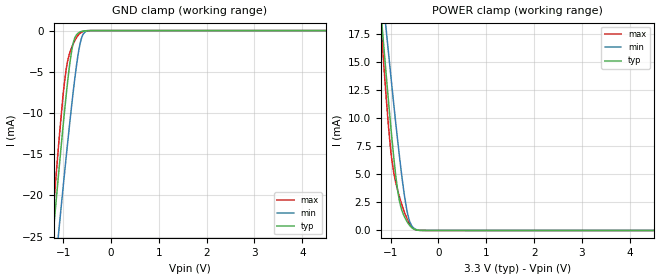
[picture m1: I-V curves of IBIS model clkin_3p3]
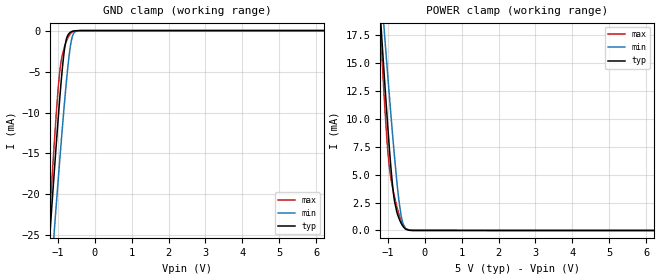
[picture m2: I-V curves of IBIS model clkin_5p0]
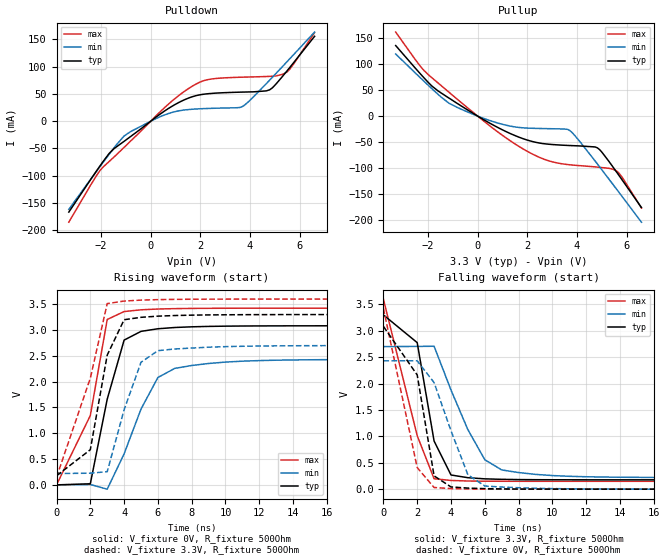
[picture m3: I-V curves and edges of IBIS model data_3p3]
| Texas Instruments Incorporated
| Small, High-Precision, Reinforced Isolated Delta-Sigma Modulator
| for Voltage Sensing Applications
| Marketing Part # : AMC3306
| Digital Voltage Range : 2.7V-5.5V
| Package-type: SOIC
| #pins/pkg drawing : 16-pin DWE
[IBIS Ver] 3.2
[File name] amc3306.ibs
[File Rev] 1.0
[Date] 08/19/2020
[Source]
| Texas Instruments Incorporated.
| 12500 TI Blvd
| Dallas, TX -75243
[Notes] Revision History:
| Rev 1.0: 08/19/2020
| - Initial version of the model
| - Model generated from simulations in SPECTRE
| - CLKIN curves from amc3306m25.ibs
| - C_comp although listed in numerical order of value are
| obtained from varying PVT conditions. For PVT conditions for
| each specific value refer the buffer description under
| respective [Model]. IBIS model user is responsible for using
| appropriate C_comp to simulate for Signal Integrity.
| - Model names with a trailing _3p3 contain the model for
| 3.3V operation. Model names with a trailing _5p0 contain the model
| for 5.0V operation.
[Disclaimer]
| This model is designed as an aid for customers of Texas Instruments.
| TI and its licensors and suppliers make no warranties, either expressed
| or implied, with respect to this model, including the warranties of
| merchantability or fitness for a particular purpose. The model is
| provided solely on an "as is" basis. The entire risk as to its quality
| and performance is with the customer.
| This model is subject to change without notice. Texas Instruments
| Incorporated is not responsible for updating this model.
[Copyright]
(C) Copyright 2020 Texas Instruments Incorporated. All rights reserved.
[Component] AMC3306
[Manufacturer] Texas Instruments Incorporated
[Package] |SOIC (DWE) 16-pin
| variable typ min max
R_pkg 0.11 0.11 0.11
L_pkg 2.9nH 2.9nH 2.9nH
C_pkg 0.4pF 0.4pF 0.4pF
| pin number (pin name) mapping to model name
[Pin]  signal_name   model_name   R_pin L_pin C_pin
1   DCDC_OUT   NC   NA   NA   NA
2   DCDC_HGND   NC   NA   NA   NA
3   HLDO_IN   NC   NA   NA   NA
4   NC   NC   NA   NA   NA
5   HLDO_OUT   NC   NA   NA   NA
6   INP   NC   NA   NA   NA
7   INN   NC   NA   NA   NA
8   HGND   NC   NA   NA   NA
9   AGND   GND   NA   NA   NA
10   DOUT   data   NA   NA   NA
11   CLKIN   clkin   NA   NA   NA
12   VDD   POWER   NA   NA   NA
13   LDO_OUT   NC   NA   NA   NA
14   DIAG   NC   NA   NA   NA
15   DCDC_GND   NC   NA   NA   NA
16   DCDC_IN   NC   NA   NA   NA
| Model Selectors
[Model Selector] clkin
clkin_3p3   3.3V digital Input
clkin_5p0   5.0V digital Input
[Model Selector] data
data_3p3   3.3V digital Output
data_5p0   5.0V digital Output
| Models and submodels in the file (4): clkin_3p3 (Input), clkin_5p0 (Input), data_3p3 (Output), data_5p0 (Output)
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|   clkin_3p3 Model
[Model]   clkin_3p3
Model_type   Input
Vinl = 0.81
Vinh = 2.52
|   typ   min   max
C_comp   1.27pF   1.27pF   1.27pF
[Voltage Range]   3.3   2.7   3.6
[Temperature Range]   25   125   -40
[Power Clamp Reference]   3.3   2.7   3.6
[GND Clamp Reference]   0   0   0
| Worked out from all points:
|   GND clamp passes 1 mA (typ) near -0.76 V on its own axis
|   POWER clamp passes 1 mA (typ) near -0.68 V on its own axis
[GND Clamp]
|   Voltage   I(typ)   I(min)   I(max)
-3.3V     -168.5mA   -163.8mA   -187mA
-1.231V   -26.22mA   -32.85mA   -23.77mA
-1.211V   -24.92mA   -31.65mA   -22.3mA
-1.092V   -17.27mA   -24.5mA    -13.76mA
-1.003V   -11.76mA   -19.24mA   -8.012mA
-933.9mV  -7.747mA   -15.26mA   -4.63mA
-815.1mV  -2.261mA   -8.782mA   -1.974mA
-745.8mV  -780uA     -5.384mA   -1.106mA
-636.9mV  -152.3uA   -1.394mA   -283.4uA
-547.8mV  -32.09uA   -196.9uA   -56.31uA
-438.9mV  -2.267uA   -11.38uA   -3.33uA
6.6V      0A         0A         0A
[POWER Clamp]
|   Voltage   I(typ)   I(min)   I(max)
-3.3V     134.4mA    118.6mA    160mA
-1.221V   20.46mA    23.51mA    19.62mA
-1.132V   15.89mA    19.63mA    14.17mA
-1.092V   13.9mA     17.92mA    11.88mA
-983.4mV  8.68mA     13.31mA    6.622mA
-884.4mV  4.605mA    9.284mA    4.137mA
-815.1mV  2.641mA    6.627mA    3.014mA
-735.9mV  1.473mA    3.887mA    1.934mA
-656.7mV  795.8uA    1.747mA    1.055mA
-597.3mV  434.4uA    769.8uA    555uA
-488.4mV  80.75uA    131.9uA    82.36uA
6.6V      0A         0A         0A
|   clkin_5p0 Model
[Model]   clkin_5p0
Model_type   Input
Vinl = 1.35
Vinh = 3.85
|   typ   min   max
C_comp   1.27pF   1.27pF   1.27pF
[Voltage Range]   5   4.5   5.5
[Temperature Range]   25   125   -40
[Power Clamp Reference]   5   4.5   5.5
[GND Clamp Reference]   0   0   0
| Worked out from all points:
|   GND clamp passes 1 mA (typ) near -0.76 V on its own axis
|   POWER clamp passes 1 mA (typ) near -0.68 V on its own axis
[GND Clamp]
|   Voltage   I(typ)   I(min)   I(max)
-5V       -287.4mA   -273.3mA   -323.4mA
-1.25V    -27.47mA   -34.01mA   -25.19mA
-1.235V   -26.49mA   -33.1mA    -24.07mA
-1.145V   -20.63mA   -27.65mA   -17.48mA
-1.1V     -17.76mA   -24.95mA   -14.3mA
-950mV    -8.649mA   -16.17mA   -5.277mA
-830mV    -2.776mA   -9.559mA   -2.198mA
-770mV    -1.136mA   -6.523mA   -1.378mA
-695mV    -365.7uA   -3.238mA   -637.9uA
-605mV    -90.88uA   -751.5uA   -166.7uA
-395mV    -749.7nA   -3.614uA   -858.5nA
10V       0A         0A         0A
[POWER Clamp]
|   Voltage   I(typ)   I(min)   I(max)
-5V       319.9mA    231.9mA    422.9mA
-1.25V    21.97mA    24.79mA    21.45mA
-1.13V    15.79mA    19.55mA    14.06mA
-1.085V   13.54mA    17.61mA    11.48mA
-995mV    9.213mA    13.8mA     7.066mA
-935mV    6.564mA    11.32mA    5.171mA
-830mV    2.979mA    7.184mA    3.241mA
-725mV    1.364mA    3.549mA    1.802mA
-635mV    651.4uA    1.322mA    855.8uA
-575mV    330.5uA    547.9uA    411.1uA
-500mV    101.7uA    162.3uA    107.5uA
10V       0A         0A         0A
|   data_3p3 Model
[Model]   data_3p3
Model_type   Output
Polarity   Non-Inverting
Vmeas = 1.65
Vref = 0
Cref = 2pF
Rref = 100000
|   typ   min   max
|   (nom PVT)   (fast PVT)   (slow PVT)
C_comp   1.01pF   1.01pF   1.27pF
| Where Nom  PVT is Nominal Process, 3.3V, 27C
|   Fast PVT is Strong Process,  3.6V, -40C
|   Slow PVT is Weak Process,   2.7V, 125C
[Voltage Range]   3.3   2.7   3.6
[Temperature Range]   25   125   -40
[Pullup Reference]   3.3   2.7   3.6
[Pulldown Reference]   0   0   0
[Power Clamp Reference]   3.3   2.7   3.6
[GND Clamp Reference]   0   0   0
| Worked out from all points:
|   slope of the pulldown table from 0 to 0.495 V, typ, clamps not added: 29.6 ohm
|   slope of the pullup table from 0 to 0.495 V, typ, clamps not added: 36.1 ohm
|   falling waveform, V_fixture 3.3V, R_fixture 500Ohm: 20-80 % time 1.12ns typ, 2.12ns min, 1.68ns max; typ from 3.3 V to 0.177 V
|   rising waveform, V_fixture 0V, R_fixture 500Ohm: 20-80 % time 1.34ns typ, 1.95ns min, 1.73ns max; typ from 0 V to 3.08 V
|   rising waveform, V_fixture 3.3V, R_fixture 500Ohm: 20-80 % time 1.17ns typ, 1.43ns min, 1.86ns max; typ from 0.177 V to 3.3 V
|   falling waveform, V_fixture 0V, R_fixture 500Ohm: 20-80 % time 1.47ns typ, 1.66ns min, 1.36ns max; typ from 3.08 V to 0 V
[Pulldown]
|   Voltage   I(typ)   I(min)   I(max)
-3.3V     -166.8mA   -161.8mA   -185.3mA
-2.043V   -81.98mA   -83.13mA   -90.47mA
-1.676V   -59.32mA   -60.73mA   -74.01mA
-1.073V   -36.93mA   -27.18mA   -48.07mA
254.1mV   8.882mA    5.691mA    11.67mA
1.125V    34.18mA    18.93mA    46.91mA
2.165V    49.66mA    23.11mA    74.74mA
3.689V    53.36mA    26.82mA    80.74mA
4.788V    57.51mA    75.23mA    82.22mA
5.481V    91.83mA    108.7mA    89.89mA
5.768V    108mA      122.7mA    105.8mA
6.6V      155.7mA    163.5mA    162.6mA
[Pullup]
|   Voltage   I(typ)   I(min)   I(max)
-3.3V     135.2mA    119.1mA    161.1mA
-2.171V   73.94mA    67.33mA    87.95mA
-1.152V   34.46mA    24.64mA    45.67mA
-676.5mV  19.94mA    13.54mA    26.63mA
838.2mV   -22.5mA    -13.7mA    -31.3mA
1.917V    -44.75mA   -22.84mA   -65.38mA
2.788V    -53.64mA   -24.1mA    -84.65mA
3.709V    -56.48mA   -27.59mA   -93.4mA
4.828V    -61.04mA   -92.09mA   -97.94mA
5.59V     -106.9mA   -139.8mA   -105mA
5.848V    -124.2mA   -156mA     -119.2mA
6.6V      -175.5mA   -203.6mA   -176.4mA
[Ramp]
R_load = 500
|   typ   min   max
dV/dt_r   1.84949/1.34068e-09   1.45841/2.16584e-09   2.05426/1.73074e-09
dV/dt_f   1.87387/1.11692e-09   1.48826/3.31067e-09   2.07072/1.67969e-09
[Falling Waveform]
V_fixture = 3.3V
V_fixture_min = 2.7V
V_fixture_max = 3.6V
R_fixture = 500Ohm
C_fixture = 0F
|   Time   V(typ)   V(min)   V(max)
0s        3.3V       2.7V       3.6V
2ns       2.775V     2.703V     1.013V
3ns       911mV      2.707V     197.4mV
4ns       268.5mV    1.877V     164.8mV
5ns       217.2mV    1.127V     154.4mV
6ns       195.5mV    557.6mV    150.8mV
7ns       186mV      364.4mV    149.6mV
9ns       179.3mV    280mV      148.9mV
17ns      176.9mV    221.3mV    148.8mV
100ns     176.9mV    219.6mV    148.8mV
[Rising Waveform]
V_fixture = 0V
V_fixture_min = 0V
V_fixture_max = 0V
R_fixture = 500Ohm
C_fixture = 0F
|   Time   V(typ)   V(min)   V(max)
0s        15.65nV    51.68nV    5.017nV
2ns       21.13mV    7.321mV    1.344V
3ns       1.66V      -83.06mV   3.204V
4ns       2.805V     601.6mV    3.358V
5ns       2.974V     1.469V     3.392V
6ns       3.025V     2.081V     3.407V
7ns       3.049V     2.257V     3.415V
10ns      3.075V     2.379V     3.422V
19ns      3.082V     2.429V     3.424V
100ns     3.082V     2.431V     3.424V
[Rising Waveform]
V_fixture = 3.3V
V_fixture_min = 2.7V
V_fixture_max = 3.6V
R_fixture = 500Ohm
C_fixture = 0F
|   Time   V(typ)   V(min)   V(max)
0s        176.9mV    219.6mV    148.8mV
2ns       681.2mV    226.3mV    2.067V
3ns       2.514V     255.6mV    3.512V
4ns       3.2V       1.455V     3.562V
5ns       3.246V     2.375V     3.58V
6ns       3.269V     2.6V       3.589V
9ns       3.293V     2.668V     3.598V
12ns      3.298V     2.69V      3.6V
18ns      3.3V       2.699V     3.6V
100ns     3.3V       2.7V       3.6V
[Falling Waveform]
|Gnd
V_fixture = 0V
V_fixture_min = 0V
V_fixture_max = 0V
R_fixture = 500Ohm
C_fixture = 0F
|   Time   V(typ)   V(min)   V(max)
0s        3.082V     2.431V     3.424V
2ns       2.164V     2.431V     408.8mV
3ns       251.2mV    2.018V     31.3mV
4ns       42.27mV    1.107V     10.94mV
5ns       20.6mV     272.2mV    3.915mV
6ns       9.81mV     59.91mV    1.425mV
9ns       1.283mV    17.31mV    93.35uV
15ns      24.86uV    1.194mV    667.5nV
100ns     21.94nV    63.49nV    3.768nV
